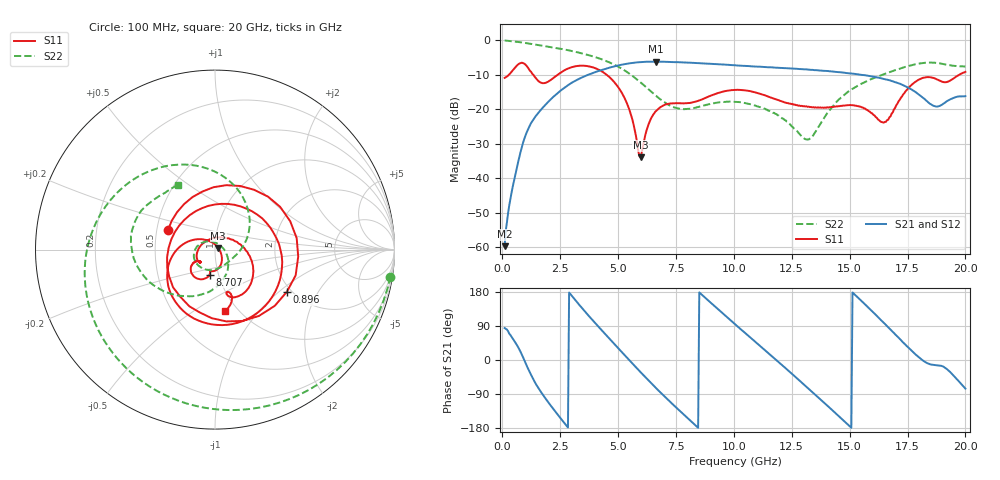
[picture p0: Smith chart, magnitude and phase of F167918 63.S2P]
!  2-Port S-parameters saved by WinCal
! VAR MeasName=S-Parameters (CALIBRATED_DATA) read from VNA (N5242A)
! VAR MeasDate=2016-11-22 10:27:58
! VAR NAME=F167918 63
! VAR FILENAME=F167918 63.S2P
! VAR DATE=2016-11-22 10:27:58
! VAR PHYS_PORTS=1,2
# Hz S DB R 50
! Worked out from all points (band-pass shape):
!   401 points, 100 MHz to 20 GHz, reference 50 ohm
!   highest |S21| = -6.22 dB at 6.617 GHz (marker M1); lowest = -59.7 dB at 100 MHz (marker M2)
!   |S21| within 3 dB of the highest: 4.033 GHz to 14.43 GHz (10.4 GHz wide, 113 % of centre)
!   lowest |S11| = -33.9 dB at 5.971 GHz (marker M3), VSWR 1.04, Z = 51.8 + j0.94 ohm
!   |S11| at or under -10 dB: start of sweep to 290.2 MHz; 1.335 GHz to 2.392 GHz (1.057 GHz wide, 56.7 % of centre); 4.499 GHz to 19.74 GHz (15.24 GHz wide, 126 % of centre)
!   |S22| runs from -28.8 to -0.1 dB; largest |S21 - S12| = 0.004
!   S11 on the Smith chart (normalised r, x): 100 MHz: 0.57, +0.14; 896 MHz: 1.89, -1.13; 8.707 GHz: 0.91, -0.26; 20 GHz: 0.87, -0.68
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1e8  -10.93 157.6  -59.69 84.4  -59.41 86.9  -0.10 -8.8
5.4775e8  -8.00 57.0  -39.40 47.6  -39.52 47.7  -0.41 -44.8
8.96e8  -6.66 -30.4  -29.75 7.3  -29.82 7.7  -0.73 -70.7
1.14475e9  -8.35 -92.8  -25.37 -27.0  -25.39 -26.5  -0.98 -87.8
1.44325e9  -10.96 -160.1  -22.01 -62.6  -21.99 -62.3  -1.30 -106.7
2.13975e9  -11.31 66.7  -16.86 -124.1  -16.86 -124.0  -2.06 -145.5
2.7865e9  -8.37 -10.7  -13.28 -174.3  -13.27 -174.0  -2.84 -176.9
3.43325e9  -7.39 -68.8  -10.83 137.7  -10.79 138.0  -3.83 154.2
4.279e9  -8.99 -131.6  -8.67 79.5  -8.60 79.3  -5.52 117.4
5.02525e9  -13.81 177.5  -7.30 29.9  -7.29 29.5  -7.76 83.2
5.9705e9  -33.93 26.8  -6.36 -31.9  -6.38 -32.1  -12.22 37.8
6.61725e9  -20.67 -70.3  -6.22 -72.6  -6.23 -72.6  -16.00 7.4
6.7665e9  -19.75 -77.7  -6.23 -81.7  -6.24 -81.8  -16.84 0.1
7.81125e9  -18.32 -102.8  -6.46 -142.8  -6.44 -142.6  -19.98 -50.7
8.70675e9  -16.95 -102.4  -6.74 167.3  -6.73 167.3  -18.93 -94.5
1.005e10  -14.42 -123.9  -7.27 94.5  -7.26 94.5  -17.88 -149.7
1.169175e10  -16.88 -147.9  -7.92 7.4  -7.89 7.2  -21.05 159.0
1.338325e10  -19.49 -142.3  -8.60 -84.3  -8.57 -84.3  -27.93 26.3
1.5025e10  -18.81 -146.3  -9.65 -176.1  -9.64 -176.4  -14.50 -79.6
1.67165e10  -22.35 65.9  -11.61 83.5  -11.72 83.8  -9.31 -133.3
1.796025e10  -11.55 -38.2  -15.62 8.6  -15.51 9.4  -6.83 -173.8
2e10  -9.18 -80.9  -16.23 -75.5  -16.08 -75.5  -7.65 119.5
